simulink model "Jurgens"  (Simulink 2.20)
settings: Solver=ode3  StartTime=0.0  StopTime=1  FixedStep=0.001  MaxStep=0.001  RelTol=1e-3  AbsTol=1e-6

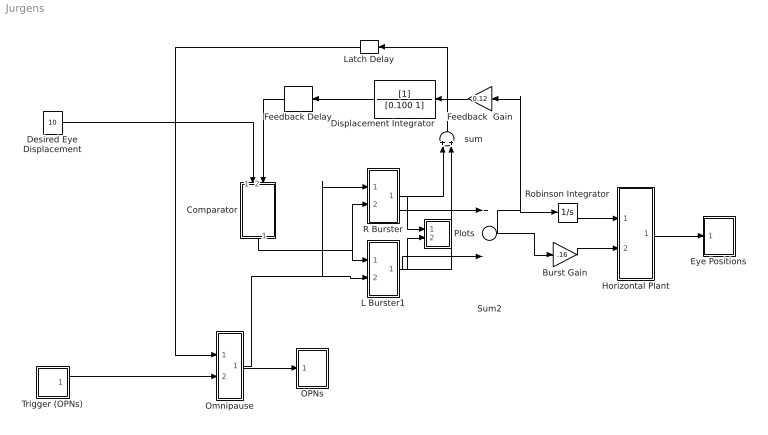
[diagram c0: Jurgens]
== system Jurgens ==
  Burst Gain : Gain  Gain=.16
  Comparator : Subsystem  Orientation=down
  Desired Eye Displacement : Constant  Value=10
  Displacement Integrator : TransferFcn  Orientation=left  Numerator=[1]  Denominator=[0.100 1]
  Eye Positions : Subsystem  mask(Graph scope.){}
      mask help: Graph scope using MATLAB graph window. Enter plotting ranges and line type.
      mask init:
      | color = @4; ax = [0, @1, @2, @3]; dt = -1;
  Feedback  Gain : Gain  Orientation=left  Gain=0.12
  Feedback Delay : TransportDelay  Orientation=left  DelayTime=.002  InitialInput=0  BufferSize=1024
  Horizontal Plant : Subsystem
  L Burster1 : Subsystem
  Latch Delay : TransportDelay  Orientation=left  DelayTime=.002  InitialInput=00  BufferSize=1024
  OPNs : Subsystem  mask(Graph scope.){}
      mask help: Graph scope using MATLAB graph window. Enter plotting ranges and line type.
      mask init:
      | color = @4; ax = [0, @1, @2, @3]; dt = -1;
  Omnipause : Subsystem
  Plots : Subsystem
  R Burster : Subsystem
  Robinson Integrator : Integrator  ExternalReset=none  InitialConditionSource=internal  InitialCondition=0  LimitOutput=off  UpperSaturationLimit=inf  LowerSaturationLimit=-inf  ShowSaturationPort=off  ShowStatePort=off  AbsoluteTolerance=auto
  Sum2 : Sum  Inputs=+-
  Trigger (OPNs) : Subsystem  mask(Pulse Generator){period=.5, duty=6, amplitude=1, start=.1}
      mask prompts: period "Period (secs):"; duty "Duty cycle (% of period):"; start "Start time:"
      mask help: Pulse Generator
  sum : Sum  Orientation=up  Inputs=++
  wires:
  Displacement Integrator/1 -> Feedback Delay/1
  Feedback Delay/1 -> Comparator/2(in_2)
  Burst Gain/1 -> Horizontal Plant/2(in_2)
  Sum2/1 -> Burst Gain/1, Robinson Integrator/1, Feedback  Gain/1
  Horizontal Plant/1(out_1) -> Eye Positions/1(x)
  Comparator/1(out_1) -> L Burster1/1(in_1), R Burster/2(in_1)
  sum/1 -> Latch Delay/1
  Latch Delay/1 -> Omnipause/1(in_1)
  Robinson Integrator/1 -> Horizontal Plant/1(in_1)
  Omnipause/1(out_1) -> L Burster1/2(in_2), R Burster/1(in_2), OPNs/1(x)
  R Burster/1(out_2) -> sum/1, Plots/1(in_1), Sum2/1
  L Burster1/1(out_1) -> Plots/2(in_2), Sum2/2, sum/2
  Desired Eye Displacement/1 -> Comparator/1(in_1)
  Trigger (OPNs)/1(out1) -> Omnipause/2(in_2)
  Feedback  Gain/1 -> Displacement Integrator/1

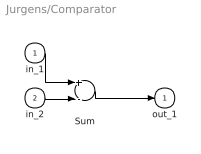
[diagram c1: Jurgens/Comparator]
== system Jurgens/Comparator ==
  in_1 : Inport  Port=1  PortWidth=-1  SampleTime=-1
  in_2 : Inport  Port=2  PortWidth=-1  SampleTime=-1
  Sum : Sum  Inputs=+-
  out_1 : Outport  Port=1  InitialOutput=0
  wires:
  Sum/1 -> out_1/1
  in_1/1 -> Sum/1
  in_2/1 -> Sum/2

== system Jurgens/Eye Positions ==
  x : Inport  Port=1  PortWidth=-1  SampleTime=-1
  "S-function M-file which plots lines " : S-Function  FunctionName=sfuny  Parameters=ax, color,dt  PortCounts=[]  SFunctionModules=''
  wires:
  x/1 -> "S-function M-file which plots lines "/1

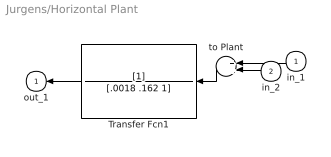
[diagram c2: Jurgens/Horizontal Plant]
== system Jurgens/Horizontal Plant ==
  in_1 : Inport  Orientation=left  Port=1  PortWidth=-1  SampleTime=-1
  in_2 : Inport  Orientation=left  Port=2  PortWidth=-1  SampleTime=-1
  Transfer Fcn1 : TransferFcn  Orientation=left  Numerator=[1]  Denominator=[.0018 .162 1]
  to Plant : Sum  Orientation=left  Inputs=++
  out_1 : Outport  Orientation=left  Port=1  InitialOutput=0
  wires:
  to Plant/1 -> Transfer Fcn1/1
  in_1/1 -> to Plant/1
  in_2/1 -> to Plant/2
  Transfer Fcn1/1 -> out_1/1

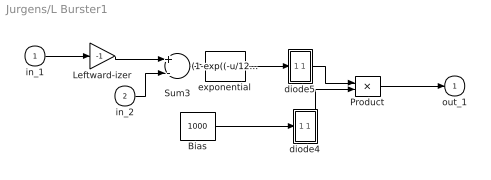
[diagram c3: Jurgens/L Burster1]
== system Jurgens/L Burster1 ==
  in_1 : Inport  Port=1  PortWidth=-1  SampleTime=-1
  in_2 : Inport  Port=2  PortWidth=-1  SampleTime=-1
  Bias : Constant  Value=1000
  Leftward-izer : Gain  Gain=-1
  Product : Product  Inputs=2
  Sum3 : Sum  Inputs=+-
  diode4 : Subsystem
  diode5 : Subsystem
  exponential : Fcn  Expr=(1-exp((-u/12)))
  out_1 : Outport  Port=1  InitialOutput=0
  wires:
  Product/1 -> out_1/1
  in_2/1 -> Sum3/2
  Sum3/1 -> exponential/1
  Bias/1 -> diode4/1(in_1)
  diode5/1(out_1) -> Product/1
  exponential/1 -> diode5/1(in_1)
  diode4/1(out_1) -> Product/2
  in_1/1 -> Leftward-izer/1
  Leftward-izer/1 -> Sum3/1

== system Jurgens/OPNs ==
  x : Inport  Port=1  PortWidth=-1  SampleTime=-1
  "S-function M-file which plots lines " : S-Function  FunctionName=sfuny  Parameters=ax, color,dt  PortCounts=[]  SFunctionModules=''
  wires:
  x/1 -> "S-function M-file which plots lines "/1

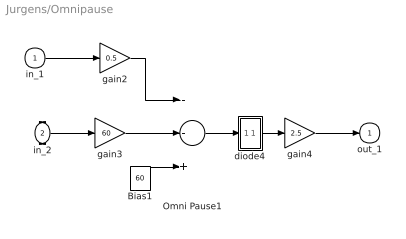
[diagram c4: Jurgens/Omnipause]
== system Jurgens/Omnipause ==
  in_1 : Inport  Port=1  PortWidth=-1  SampleTime=-1
  in_2 : Inport  Port=2  PortWidth=-1  SampleTime=-1
  Bias1 : Constant  Value=60
  Omni Pause1 : Sum  Inputs=--+
  diode4 : Subsystem
  gain2 : Gain  Gain=0.5
  gain3 : Gain  Gain=60
  gain4 : Gain  Gain=2.5
  out_1 : Outport  Port=1  InitialOutput=0
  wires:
  Omni Pause1/1 -> diode4/1(in_1)
  Bias1/1 -> Omni Pause1/3
  in_1/1 -> gain2/1
  gain2/1 -> Omni Pause1/1
  diode4/1(out_1) -> gain4/1
  gain4/1 -> out_1/1
  in_2/1 -> gain3/1
  gain3/1 -> Omni Pause1/2

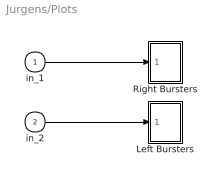
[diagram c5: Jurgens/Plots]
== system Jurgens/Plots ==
  in_1 : Inport  Port=1  PortWidth=-1  SampleTime=-1
  in_2 : Inport  Port=2  PortWidth=-1  SampleTime=-1
  Left Bursters : Subsystem  mask(Graph scope.){}
      mask help: Graph scope using MATLAB graph window. Enter plotting ranges and line type.
      mask init:
      | color = @4; ax = [0, @1, @2, @3]; dt = -1;
  Right Bursters : Subsystem  mask(Graph scope.){}
      mask help: Graph scope using MATLAB graph window. Enter plotting ranges and line type.
      mask init:
      | color = @4; ax = [0, @1, @2, @3]; dt = -1;
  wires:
  in_1/1 -> Right Bursters/1(x)
  in_2/1 -> Left Bursters/1(x)

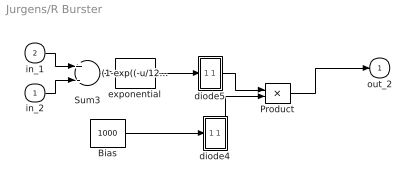
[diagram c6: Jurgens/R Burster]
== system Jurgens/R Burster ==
  in_2 : Inport  Port=1  PortWidth=-1  SampleTime=-1
  in_1 : Inport  Port=2  PortWidth=-1  SampleTime=-1
  Bias : Constant  Value=1000
  Product : Product  Inputs=2
  Sum3 : Sum  Inputs=+-
  diode4 : Subsystem
  diode5 : Subsystem
  exponential : Fcn  Expr=(1-exp((-u/12)))
  out_2 : Outport  Port=1  InitialOutput=0
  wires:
  diode4/1(out_1) -> Product/2
  Product/1 -> out_2/1
  exponential/1 -> diode5/1(in_1)
  diode5/1(out_1) -> Product/1
  in_1/1 -> Sum3/1
  in_2/1 -> Sum3/2
  Bias/1 -> diode4/1(in_1)
  Sum3/1 -> exponential/1

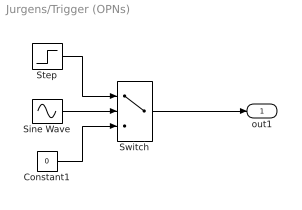
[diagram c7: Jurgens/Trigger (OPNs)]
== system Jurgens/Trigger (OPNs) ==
  Constant1 : Constant  Value=0
  Sine Wave : Sin  Amplitude=1  Frequency=2*pi./period  Phase=-2*pi*(start./period + duty/200 - 1/4)  SampleTime=-1
  Step : Step  Time=start  Before=0  After=amplitude
  Switch : Switch  Threshold=sin(pi*(0.5 - duty/100))
  out1 : Outport  Port=1  InitialOutput=0
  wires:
  Step/1 -> Switch/1
  Constant1/1 -> Switch/3
  Switch/1 -> out1/1
  Sine Wave/1 -> Switch/2

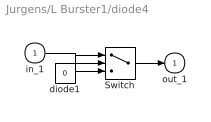
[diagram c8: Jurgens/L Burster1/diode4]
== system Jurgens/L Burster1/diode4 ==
  in_1 : Inport  Port=1  PortWidth=-1  SampleTime=-1
  Switch : Switch  Threshold=0
  diode1 : Constant  Value=0
  out_1 : Outport  Port=1  InitialOutput=0
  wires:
  in_1/1 -> Switch/2, Switch/1
  Switch/1 -> out_1/1
  diode1/1 -> Switch/3

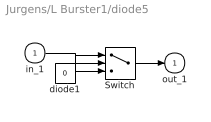
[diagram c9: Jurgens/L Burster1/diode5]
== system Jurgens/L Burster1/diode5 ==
  in_1 : Inport  Port=1  PortWidth=-1  SampleTime=-1
  Switch : Switch  Threshold=0
  diode1 : Constant  Value=0
  out_1 : Outport  Port=1  InitialOutput=0
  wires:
  diode1/1 -> Switch/3
  Switch/1 -> out_1/1
  in_1/1 -> Switch/2, Switch/1

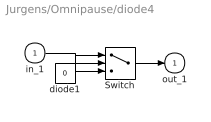
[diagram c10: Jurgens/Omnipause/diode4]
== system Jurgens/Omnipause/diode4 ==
  in_1 : Inport  Port=1  PortWidth=-1  SampleTime=-1
  Switch : Switch  Threshold=0
  diode1 : Constant  Value=0
  out_1 : Outport  Port=1  InitialOutput=0
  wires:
  diode1/1 -> Switch/3
  Switch/1 -> out_1/1
  in_1/1 -> Switch/1, Switch/2

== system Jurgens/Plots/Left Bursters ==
  x : Inport  Port=1  PortWidth=-1  SampleTime=-1
  "S-function M-file which plots lines " : S-Function  FunctionName=sfuny  Parameters=ax, color,dt  PortCounts=[]  SFunctionModules=''
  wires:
  x/1 -> "S-function M-file which plots lines "/1

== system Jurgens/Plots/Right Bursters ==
  x : Inport  Port=1  PortWidth=-1  SampleTime=-1
  "S-function M-file which plots lines " : S-Function  FunctionName=sfuny  Parameters=ax, color,dt  PortCounts=[]  SFunctionModules=''
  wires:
  x/1 -> "S-function M-file which plots lines "/1

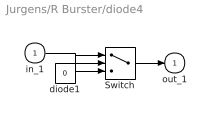
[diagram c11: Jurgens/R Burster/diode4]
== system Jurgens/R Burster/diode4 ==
  in_1 : Inport  Port=1  PortWidth=-1  SampleTime=-1
  Switch : Switch  Threshold=0
  diode1 : Constant  Value=0
  out_1 : Outport  Port=1  InitialOutput=0
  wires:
  diode1/1 -> Switch/3
  Switch/1 -> out_1/1
  in_1/1 -> Switch/1, Switch/2

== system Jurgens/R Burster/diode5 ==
  in_1 : Inport  Port=1  PortWidth=-1  SampleTime=-1
  Switch : Switch  Threshold=0
  diode1 : Constant  Value=0
  out_1 : Outport  Port=1  InitialOutput=0
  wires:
  in_1/1 -> Switch/1, Switch/2
  Switch/1 -> out_1/1
  diode1/1 -> Switch/3
